(* Logix 5000 AddOnInstructionDefinition export ACS_VELOCITY_MOVE; software revision 24.00 *)

ADD_ON_INSTRUCTION ACS_VELOCITY_MOVE   (* revision 1.0, vendor Tolomatic, Inc. *)
VAR_INPUT
   Acceleration : REAL; {required}   // Trajectory Acceleration
   Deceleration : REAL; {required}   // Trajectory Deceleration
   Velocity : REAL; {required}   // Trajectory Constance Velocity
   Force : REAL; {required}   // Force Limit (Percent)
END_VAR
VAR_IN_OUT
   DriveMoveSelect : SINT; {required}   // ACS.O.MOVESELECT
   DriveTargetAcc : REAL; {required}   // ACS.O.TARGET_0_ACC
   DriveTargetDec : REAL; {required}   // ACS.O.TARGET_0_DEC
   DriveTargetForce : REAL; {required}   // ACS.O.TARGET_0_FORCE
   DriveTargetMotionType : DINT; {required}   // ACS.O.TARGET_0_MOTION_TYPE
   DriveTargetPos : REAL; {required}   // ACS.O.TARGET_0_POS
   DriveTargetVel : REAL; {required}   // ACS.O.TARGET_0_VEL
END_VAR
VAR
   AbsVelocity : REAL; {access None}   // Absolute Value of Velocity Input
END_VAR

ROUTINE Logic   (* ladder *)
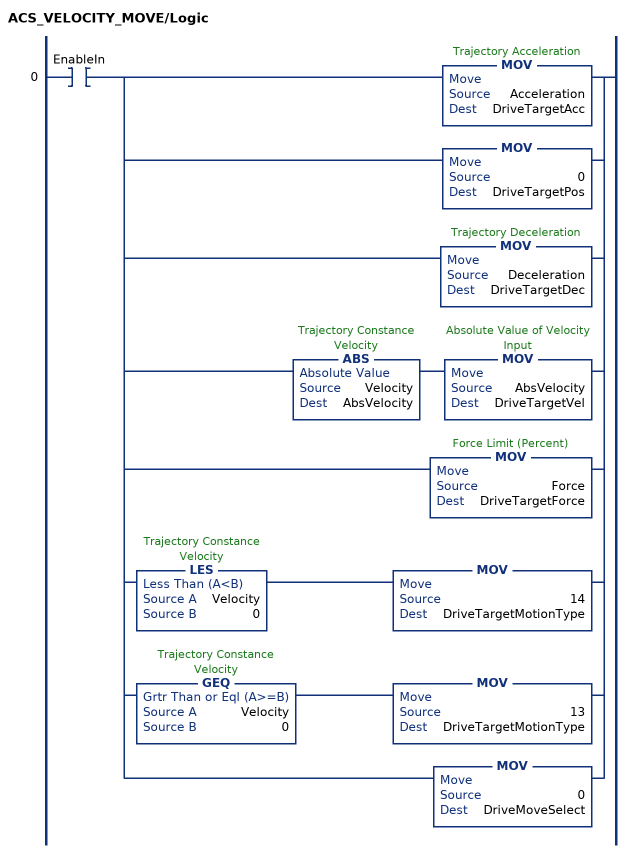
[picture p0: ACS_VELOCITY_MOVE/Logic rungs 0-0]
   0: XIC(EnableIn)[MOV(Acceleration,DriveTargetAcc) ,MOV(0,DriveTargetPos) ,MOV(Deceleration,DriveTargetDec) ,ABS(Velocity,AbsVelocity) MOV(AbsVelocity,DriveTargetVel) ,MOV(Force,DriveTargetForce) ,LES(Velocity,0) MOV(14,DriveTargetMotionType) ,GEQ(Velocity,0) MOV(13,DriveTargetMotionType) ,MOV(0,DriveMoveSelect) ];
END_ROUTINE
END_ADD_ON_INSTRUCTION
